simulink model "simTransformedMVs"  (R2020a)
settings: Solver=ode15s  StartTime=0.0  StopTime=tsim  MaxStep=1  RelTol=1e-3
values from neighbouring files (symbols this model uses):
  d1_step = 25    [runTransformedMVs.m]
  d1_step_cb = d1stepcb(n)    [runTransformedMVs.m]
  d1nom = T0nom    (= 10)    [runTransformedMVs.m]
  d2_step = d2nom*0.5    (= 0.005)    [runTransformedMVs.m]
  d2nom = qnom    (= 0.01)    [runTransformedMVs.m]
  Kc = 1/(tauC+theta)    (= 0.01)    [runTransformedMVs.m]
  p = [V;rho;cp;A;tau0;MV;transf]    [runTransformedMVs.m]
  tauI = 4*(tauC+theta)    (= 400)    [runTransformedMVs.m]
  Tnom = 50    [runTransformedMVs.m]
  transf = p(7)    [CalcBlock.m]    (also in runTransformedMVs.m = j)
  Tstep = 2    [runTransformedMVs.m]
  tstep_d1 = 100    [runTransformedMVs.m]
  tstep_d2 = 2000    [runTransformedMVs.m]
  tstep_T1 = 4000    [runTransformedMVs.m]
  tstep_T2 = 8000    [runTransformedMVs.m]
  umax = 3*Qnom    (= 5016)    [runTransformedMVs.m]
  vbias = 0    [runTransformedMVs.m]
  vmin = -inf    [runTransformedMVs.m]
undefined symbols (not defined in the file or in its folder): CalcBlock, Tank

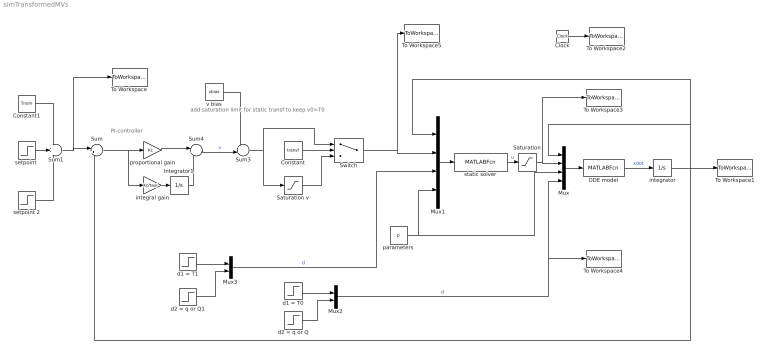
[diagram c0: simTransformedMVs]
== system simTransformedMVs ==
  note: add saturation limit for static transf to keep v0>T0
  note: PI-controller
  " integrator" : Integrator  InitialCondition=Tnom
  Clock : Clock
  Constant : Constant  Value=transf
  Constant1 : Constant  Value=Tnom
  Integrator1 : Integrator
  Mux : Mux
  Mux1 : Mux
  Mux2 : Mux  Inputs=2
  Mux3 : Mux  Inputs=2
  ODE model : MATLABFcn  MATLABFcn=Tank(u(1), u(2),u(3:9),u(10:11))  OutputDimensions=1
  Saturation : Saturate  UpperLimit=umax  LowerLimit=0
  Saturation v : Saturate  UpperLimit=inf  LowerLimit=vmin
  Sum : Sum  Inputs=|+-
  Sum1 : Sum  Inputs=+++
  Sum3 : Sum  Inputs=++|
  Sum4 : Sum  Inputs=|++
  Switch : Switch  Criteria=u2 ~= 0
  To Workspace : ToWorkspace  VariableName=Tsp  SampleTime=-1
  To Workspace1 : ToWorkspace  VariableName=T  SampleTime=-1
  To Workspace2 : ToWorkspace  VariableName=time  SampleTime=-1
  To Workspace3 : ToWorkspace  VariableName=u  SampleTime=-1
  To Workspace4 : ToWorkspace  VariableName=d  SampleTime=-1
  To Workspace5 : ToWorkspace  VariableName=v  SampleTime=-1
  d1 = T0 : Step  Time=tstep_d1  Before=d1nom  After=d1_step  SampleTime=0
  d1 = T1 : Step  Time=tstep_d1  Before=d1nom  After=d1_step_cb  SampleTime=0
  d2 = q or Q : Step  Time=tstep_d2  Before=d2nom  After=d2_step  SampleTime=0
  d2 = q or Q1 : Step  Time=tstep_d2  Before=d2nom  After=d2_step  SampleTime=0
  integral gain : Gain  Gain=Kc/tauI  Multiplication=Matrix(K*u)
  parameters : Constant  Value=p
  proportional gain : Gain  Gain=Kc  Multiplication=Matrix(K*u)
  "setpoint " : Step  Time=tstep_T1  After=Tstep  SampleTime=0
  setpoint 2 : Step  Time=tstep_T2  After=-Tstep  SampleTime=0
  static solver : MATLABFcn  MATLABFcn=CalcBlock(u(1),u(2),u(3:4),u(5:11))  OutputDimensions=1
  v bias : Constant  Value=vbias
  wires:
  " integrator"/1 -> Mux/1, Mux1/1, Sum/2, To Workspace1/1  "T"
  Mux/1 -> ODE model/1
  Clock/1 -> To Workspace2/1
  Sum/1 -> integral gain/1, proportional gain/1
  static solver/1 -> Saturation/1  "u"
  Sum4/1 -> Sum3/2  "v"
  Mux1/1 -> static solver/1
  ODE model/1 -> " integrator"/1  "xdot"
  integral gain/1 -> Integrator1/1
  proportional gain/1 -> Sum4/1
  Integrator1/1 -> Sum4/2
  Mux2/1 -> Mux/4, To Workspace4/1  "d"
  parameters/1 -> Mux/3, Mux1/4
  v bias/1 -> Sum3/1
  Sum3/1 -> Saturation v/1, Switch/1
  Saturation/1 -> Mux/2, To Workspace3/1
  Switch/1 -> Mux1/2, To Workspace5/1
  Saturation v/1 -> Switch/3
  Constant/1 -> Switch/2
  "setpoint "/1 -> Sum1/2
  Sum1/1 -> To Workspace/1, Sum/1
  setpoint 2/1 -> Sum1/3
  d1 = T0/1 -> Mux2/1
  d2 = q or Q/1 -> Mux2/2
  Constant1/1 -> Sum1/1
  d2 = q or Q1/1 -> Mux3/2
  d1 = T1/1 -> Mux3/1
  Mux3/1 -> Mux1/3  "d"
